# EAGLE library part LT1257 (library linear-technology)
Complete Single Supply 12-Bit Voltage Output DAC Source: http://www.linear.com/pc/downloadDocument.do?navId=H0,C1,C1155,C1005,C1156,P1425,D3414
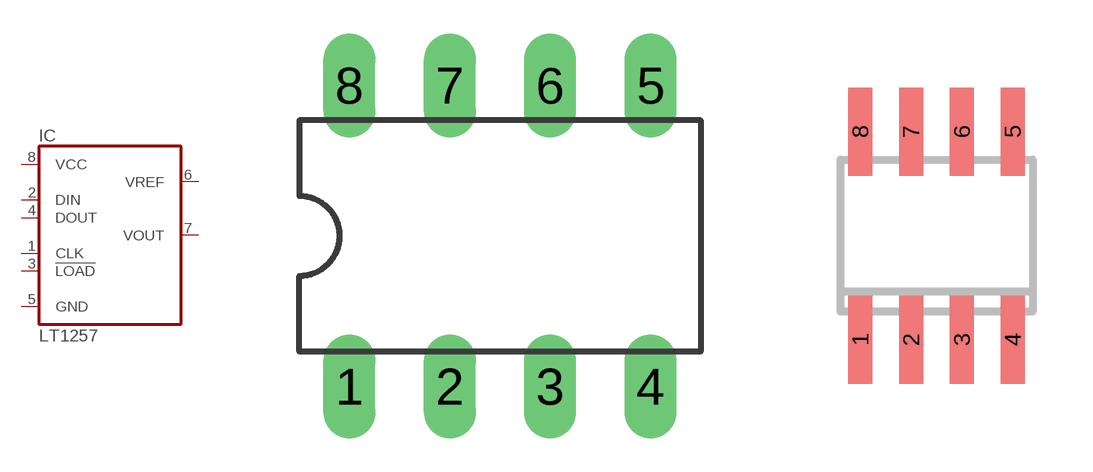
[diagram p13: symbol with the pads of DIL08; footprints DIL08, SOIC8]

Designator prefix IC

## LT1257N (OC_FARNELL: unknown; OC_NEWARK: unknown)  [DIL08]
1  CLK  in
2  DIN  in
3  !LOAD  in
4  DOUT  out
5  GND  pwr
6  VREF  in
7  VOUT  out
8  VCC  pwr

## LT1257S (OC_FARNELL: unknown; OC_NEWARK: unknown)  [SOIC8]
Pads as for DIL08

## Footprint DIL08 (pad centres in mm)
Dual In Line Package
drill 0.813 long: 1 -3.81,-3.81; 2 -1.27,-3.81; 3 1.27,-3.81; 4 3.81,-3.81; 5 3.81,3.81; 6 1.27,3.81; 7 -1.27,3.81; 8 -3.81,3.81

## Footprint SOIC8 (pad centres in mm)
Small Outline IC
smd 0.6 x 2.2: 1 -1.905,-2.6; 2 -0.635,-2.6; 3 0.635,-2.6; 4 1.905,-2.6; 5 1.905,2.6; 6 0.635,2.6; 7 -0.635,2.6; 8 -1.905,2.6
